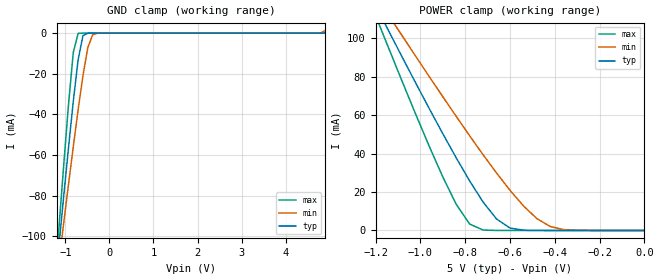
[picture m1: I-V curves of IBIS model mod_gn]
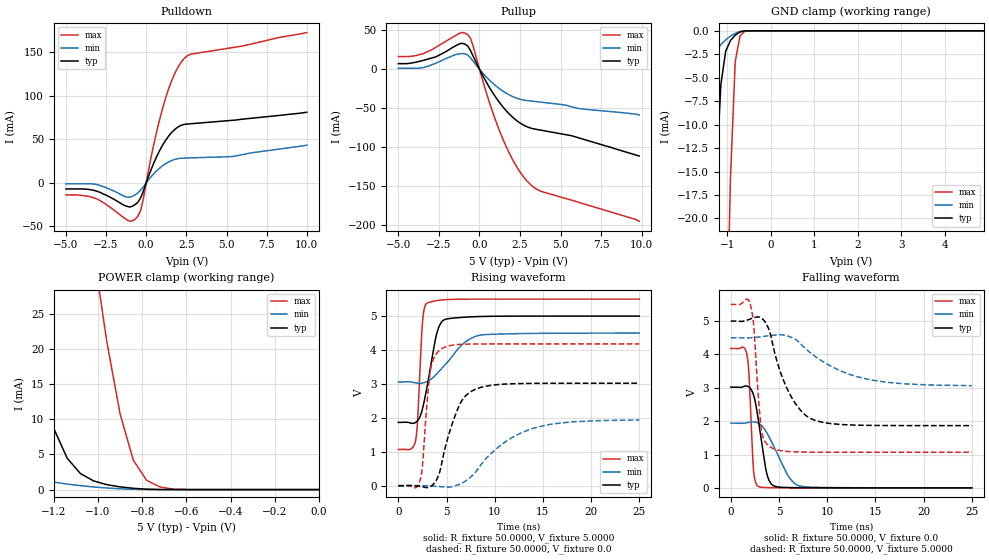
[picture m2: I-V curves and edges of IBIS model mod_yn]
| IBIS (I/O, Buffer, Information, Specification) Model, officially
| electronic behavioral standard for Buffer structures of digital pins.
[IBIS ver]  4.0
[File name] 54hc244_5v0_rev1.ibs
[File Rev]  1.0
[Date]   23 Nov 2018
[Source]   CAD & Design Services (Catania) - STMicroelectronics
[Notes]
  (Note1) This IBIS model is the model of the product with package
   (Flat20 package elements);
  (Note2) This IBIS model is extracted with nominal 5.0V power supply
   (min:4.5V, typ:5.0V, max:5.5V);
  (Note3) This model has few Warnings about the non-monotonicity
   of I-V curves, but they are not indicative of problems
   inside the model;
[Disclaimer]
   Customers are solely responsible for all aspects of their
   own product designs or applications using this IBIS Model.
   STMicroelectronics assumes no liability for Custmer Designs
   and applications associated to this IBIS Model.
   In the use of this IBIS Model Customer shall not modify,
   disassemble, alter this Model in whole or in part.
   If Customers do not accept these terms, the IBIS Model
   may not be used. For any problems or modifications please
   contact STMicroelectronics (www.st.com).
[Copyright] (c) 2018 STMicroelectronics
|   Component 54HC244
[Component] 54HC244
[Manufacturer] STMicroelectronics
[Package]
| variable  typ   min   max
R_pkg   0.0   0.0   0.0
L_pkg   0.0H   0.0H   0.0H
C_pkg   0.0F   0.0F   0.0F
[Pin]  signal_name   model_name   R_pin   L_pin   C_pin
1   1GN   mod_gn   178.9m   6.2nH   1.2pF
2   1A1   mod_an   182.5m   6.3nH   1.2pF
3   2Y4   mod_yn   114.4m   3.5nH   1.3pF
4   1A2   mod_an   79.1m   2.3nH   0.9pF
5   2Y3   mod_yn   75.8m   2.2nH   0.8pF
6   1A3   mod_an   75.8m   2.2nH   0.8pF
7   2Y2   mod_yn   84.5m   2.4nH   0.9pF
8   1A4   mod_an   116.2m   3.6nH   1.3pF
9   2Y1   mod_yn   178.9m   6.2nH   1.2pF
10   GND   GND   117.4m   4.4nH   1.2pF
11   2A1   mod_an   178.9m   6.2nH   1.2pF
12   1Y4   mod_yn   189.6m   6.6nH   1.2pF
13   2A2   mod_an   125.1m   3.9nH   1.3pF
14   1Y3   mod_yn   86.3m   2.5nH   0.9pF
15   2A3   mod_an   79.4m   2.3nH   0.8pF
16   1Y2   mod_yn   75.8m   2.2nH   0.8pF
17   2A4   mod_an   75.6m   2.1nH   0.9pF
18   1Y1   mod_yn   89.3m   2.7nH   1.3pF
19   2GN   mod_gn   184.3m   6.4nH   1.2pF
20   VCC   POWER   118.0m   4.4nH   1.2pF
| Models and submodels in the file (3): mod_gn (Input), mod_an (Input), mod_yn (3-state)
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|   Model mod_gn
[Model]   mod_gn
Model_type Input
Vinl   =   0.6500V
Vinh   =   1.2000V
C_comp   5.000pF   4.500pF   5.500pF
[Temperature Range]  25.0000   0.1250k   -55.0000
[Voltage Range]   5.0000V   4.5000V   5.5000V
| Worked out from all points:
|   GND clamp passes 1 mA (typ) near -0.58 V on its own axis
|   POWER clamp passes 1 mA (typ) near -0.59 V on its own axis
[GND_clamp]
|Voltage   I(typ)   I(min)   I(max)
-5V       -1.013A    -824.7mA   -1.262A
-1.15V    -105.6mA   -113.4mA   -97.24mA
-1.04V    -80.93mA   -93.95mA   -65.8mA
-930mV    -56.77mA   -74.74mA   -35.64mA
-820mV    -33.66mA   -55.92mA   -9.537mA
-710mV    -13.12mA   -37.77mA   -140.3uA
-600mV    -1.249mA   -20.9mA    -413.2nA
-490mV    -21.08uA   -7.141mA   -1.195nA
-380mV    -292.3nA   -775.9uA   -9.676pA
-160mV    -61.31pA   -1.448uA   -5.82pA
4.68V     4.486pA    2.583uA    3.86pA
4.9V      4.939pA    1.285mA    4.3pA
[POWER_clamp]
|Voltage   I(typ)   I(min)   I(max)
-4.98V    1.009A     821mA      1.256A
-1.2V     117mA      122.3mA    111.7mA
-1.14V    103.4mA    111.6mA    94.35mA
-1.08V    89.86mA    101mA      77.13mA
-900mV    50.33mA    69.56mA    27.86mA
-840mV    37.74mA    59.31mA    13.61mA
-780mV    25.73mA    49.23mA    3.335mA
-660mV    5.98mA     29.88mA    10.04uA
-600mV    1.249mA    20.9mA     413.2nA
-480mV    14.3uA     6.187mA    704.4pA
-420mV    1.386uA    2.045mA    35.02pA
0V        5.25pA     24.98nA    5.5pA
|   Model mod_out
[Model]   mod_yn
Model_type 3-state
Polarity   Inverting
Enable   Active-High
Vmeas  =   2.500V
Cref   =   50pF
C_comp   10.000pF   9.000pF   11.000pF
[Temperature Range]  25.0000   0.1250k   -55.0000
[Voltage Range]   5.0000V   4.5000V   5.5000V
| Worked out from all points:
|   slope of the pulldown table from 0 to 0.75 V, typ, clamps not added: 22.1 ohm
|   slope of the pullup table from 0 to 0.75 V, typ, clamps not added: 26.8 ohm
|   GND clamp passes 1 mA (typ) near -0.92 V on its own axis
|   POWER clamp passes 1 mA (typ) near -0.99 V on its own axis
|   rising waveform, R_fixture 50.0000, V_fixture 5.0000: 20-80 % time 1.21ns typ, 2.69ns min, 452ps max; typ from 1.87 V to 5 V
|   rising waveform, R_fixture 50.0000, V_fixture 0.0: 20-80 % time 1.95ns typ, 4.73ns min, 722ps max; typ from 0 V to 3.02 V
|   falling waveform, R_fixture 50.0000, V_fixture 0.0: 20-80 % time 966ps typ, 1.98ns min, 394ps max; typ from 3.02 V to 0 V
|   falling waveform, R_fixture 50.0000, V_fixture 5.0000: 20-80 % time 2.49ns typ, 5.29ns min, 649ps max; typ from 5 V to 1.87 V
[Pulldown]
|Voltage   I(typ)   I(min)   I(max)
-5V       -6.932mA   -1.113mA   -13.78mA
-3.24V    -8.632mA   -1.353mA   -17.21mA
-1.16V    -27.13mA   -16.53mA   -42.79mA
-680mV    -24.91mA   -13.67mA   -41.66mA
-360mV    -17.64mA   -8.787mA   -32.31mA
600mV     28.05mA    12.91mA    54.68mA
1.24V     49.72mA    22.4mA     99.18mA
1.72V     60.38mA    26.62mA    123.2mA
2.36V     67.13mA    28.46mA    142.7mA
2.84V     68mA       28.74mA    148mA
5.4V      71.89mA    30.36mA    155.4mA
10V       81.11mA    43.27mA    172.6mA
[Pullup]
|Voltage   I(typ)   I(min)   I(max)
-5V       7.182mA    1.213mA    16.3mA
-3.44V    11.53mA    2.324mA    20.22mA
-1.2V     32.87mA    19.89mA    46.45mA
-720mV    29.66mA    18.2mA     44.23mA
-400mV    17.18mA    10.46mA    30.46mA
560mV     -21.51mA   -12.84mA   -39.22mA
1.36V     -46.18mA   -26.96mA   -85.58mA
2.16V     -63.72mA   -36.12mA   -120.6mA
2.96V     -74.13mA   -40.31mA   -144.2mA
3.76V     -78.16mA   -42.21mA   -156.5mA
5.68V     -85.42mA   -48.19mA   -168.1mA
9.84V     -111.4mA   -58.63mA   -195.2mA
[GND_clamp]
|Voltage   I(typ)   I(min)   I(max)
-5V       -859mA     -590.7mA   -1.211A
-1.81V    -119.9mA   -30.89mA   -252.2mA
-1.7V     -96.39mA   -18.34mA   -220.1mA
-1.48V    -51.76mA   -4.928mA   -156.7mA
-1.37V    -31.87mA   -3.034mA   -125.6mA
-1.26V    -15.59mA   -2.105mA   -95.13mA
-1.15V    -5.709mA   -1.471mA   -65.79mA
-1.04V    -2.174mA   -968.6uA   -38.5mA
-930mV    -1.041mA   -566.4uA   -15.76mA
-820mV    -460.1uA   -265uA     -3.292mA
-600mV    -8.932uA   -10.27uA   -44.53uA
4.9V      5.062pA    3.048nA    4.3pA
[POWER_clamp]
|Voltage   I(typ)   I(min)   I(max)
-4.98V    854.3mA    587mA      1.205A
-1.8V     117.7mA    29.3mA     249.2mA
-1.56V    67.27mA    7.197mA    179.5mA
-1.38V    33.21mA    2.37mA     128.3mA
-1.32V    23.49mA    1.791mA    111.5mA
-1.2V     8.665mA    1.055mA    78.84mA
-1.14V    4.486mA    788.3uA    63.05mA
-1.02V    1.236mA    378.8uA    33.73mA
-960mV    702.2uA    228.8uA    21.01mA
-840mV    186.3uA    40.51uA    4.171mA
-780mV    61.14uA    11.93uA    1.328mA
0V        6.121pA    17.78pA    6.5pA
[Ramp]
| variable   typ   min   max
dV/dt_r   1.8152/1.9904n   1.1633/5.0618n   2.5077/0.8044n
dV/dt_f   1.8784/2.5788n   0.8617/5.1074n   2.6591/0.7414n
R_load = 50.0000
[Rising Waveform]
R_fixture= 50.0000
V_fixture= 5.0000
V_fixture_min= 4.5000
V_fixture_max= 5.5000
|time   V(typ)   V(min)   V(max)
0s        1.866V     3.056V     1.068V
1.225ns   1.851V     3.062V     1.068V
1.775ns   1.862V     3.032V     1.307V
1.975ns   1.911V     3.022V     1.802V
2.525ns   2.287V     3.025V     4.873V
2.975ns   2.902V     3.069V     5.38V
3.975ns   4.472V     3.293V     5.455V
4.825ns   4.899V     3.558V     5.482V
8.425ns   4.987V     4.435V     5.5V
25ns      5V         4.5V       5.5V
[Rising Waveform]
R_fixture= 50.0000
V_fixture= 0.0
V_fixture_min= 0.0
V_fixture_max= 0.0
|time   V(typ)   V(min)   V(max)
0s        82.21pV    127.4pV    53.46pV
2.275ns   -19.13mV   415.4uV    171.6mV
2.525ns   -31.64mV   -1.316mV   640.6mV
2.925ns   -58.11mV   -5.257mV   2.255V
3.325ns   -26.35mV   -11.1mV    3.397V
4.525ns   688.5mV    -31.62mV   4.042V
6.425ns   2.426V     50.86mV    4.165V
8.025ns   2.844V     404.1mV    4.177V
13.88ns   3.016V     1.679V     4.179V
25ns      3.02V      1.936V     4.179V
[Falling Waveform]
R_fixture= 50.0000
V_fixture= 0.0
V_fixture_min= 0.0
V_fixture_max= 0.0
|time   V(typ)   V(min)   V(max)
0s        3.02V      1.941V     4.179V
1.7ns     3.052V     1.954V     3.962V
1.9ns     3.022V     1.966V     3.34V
2.35ns    2.797V     1.978V     578.2mV
2.85ns    2.06V      1.941V     47.25mV
3.75ns    415.8mV    1.647V     8.377mV
4.6ns     46.17mV    1.161V     3.312mV
6ns       9.937mV    342mV      797.8uV
7.2ns     4.834mV    56.03mV    241.4uV
25ns      452nV      126.9uV    12.26nV
[Falling Waveform]
R_fixture= 50.0000
V_fixture= 5.0000
V_fixture_min= 4.5000
V_fixture_max= 5.5000
|time   V(typ)   V(min)   V(max)
0s        5V         4.5V       5.5V
2.075ns   5.07V      4.499V     5.451V
2.375ns   5.098V     4.507V     4.891V
2.825ns   5.127V     4.52V      2.877V
3.175ns   5.092V     4.533V     1.752V
4.125ns   4.6V       4.567V     1.221V
5.975ns   2.897V     4.547V     1.09V
8.475ns   2.055V     4.003V     1.07V
14.65ns   1.873V     3.232V     1.068V
25ns      1.866V     3.064V     1.068V
